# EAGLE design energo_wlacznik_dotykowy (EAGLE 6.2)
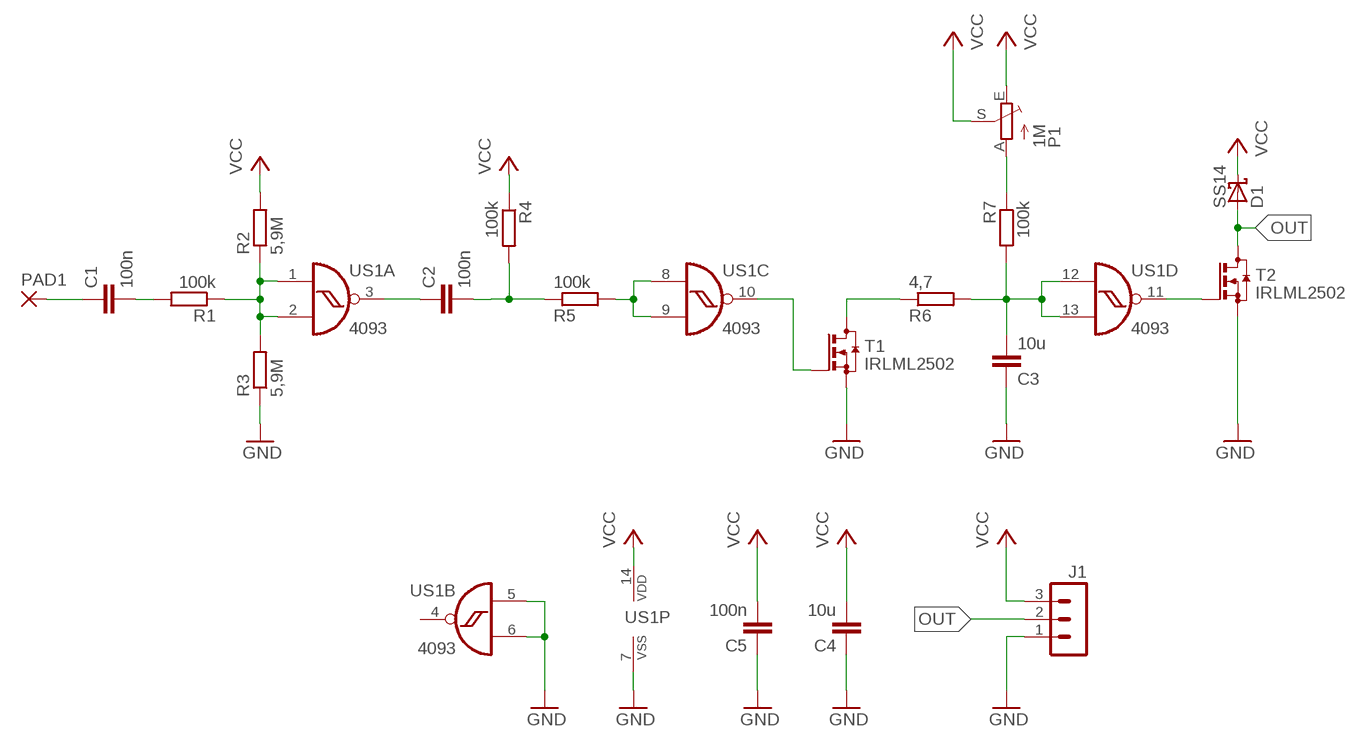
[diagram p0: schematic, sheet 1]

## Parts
C1  100n  C-EUC0805  [C0805]
C2  100n  C-EUC0805  [C0805]
C3  10u  C-EUC0805  [C0805]
C4  10u  C-EUC0805  [C0805]
C5  100n  C-EUC0805  [C0805]
D1  SS14  SCHOTTKY-DIODESMD  [SMB]
J1  MA03-1  [MA03-1]
P1  1M  TRIM_EU-CA6V  [CA6V]
PAD1  3,81/1,4  [3,81/1,4]
R1  100k  R-EU_M0805  [M0805]
R2  5,9M  R-EU_M0805  [M0805]
R3  5,9M  R-EU_M0805  [M0805]
R4  100k  R-EU_M0805  [M0805]
R5  100k  R-EU_M0805  [M0805]
R6  4,7  R-EU_M0805  [M0805]
R7  100k  R-EU_M0805  [M0805]
T1  IRLML2502  BSS123  [SOT23]
T2  IRLML2502  BSS123  [SOT23]
US1  4093  4093D  [SO14]

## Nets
GND: C3.1 C4.1 C5.1 J1.1 R3.1 T1.2(S) T2.2(S) US1.5(B:I0) US1.6(B:I1) US1.7(P:VSS)
N$1: C1.1 PAD1.1(P)
N$2: R1.1 R2.1 R3.2 US1.1(A:I0) US1.2(A:I1)
N$3: C1.2 R1.2
N$4: C2.1 US1.3(A:O)
N$5: C2.2 R4.2 R5.1
N$9: C3.2 R6.2 R7.2 US1.12(D:I0) US1.13(D:I1)
N$10: P1.A R7.1
N$11: T1.1(G) US1.10(C:O)
N$12: R6.1 T1.3(D)
N$13: T2.1(G) US1.11(D:O)
N$14: R5.2 US1.8(C:I0) US1.9(C:I1)
OUT: D1.A J1.2 T2.3(D)
VCC: C4.2 C5.2 D1.C J1.3 P1.E P1.S R2.2 R4.1 US1.14(P:VDD)
Unconnected: US1.4(B:O)

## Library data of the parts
C1-C5 = rcl:C-EU: CAPACITOR, European symbol
D1 = diode:SCHOTTKY-DIODE: Schottky Diode
J1 = con-lstb:MA03-1: PIN HEADER; OC_FARNELL: unknown; OC_NEWARK: unknown
P1 = pot:TRIM_EU-: POTENTIOMETER
PAD1 = wirepad:3,81/1,4: THROUGH-HOLE PAD
R1-R7 = rcl:R-EU_: RESISTOR, European symbol
T1 T2 = transistor-small-signal:BSS123: N-CHANNEL MOS FET
US1 = 40xx:4093: Quad 2-input NAND schmitt trigger

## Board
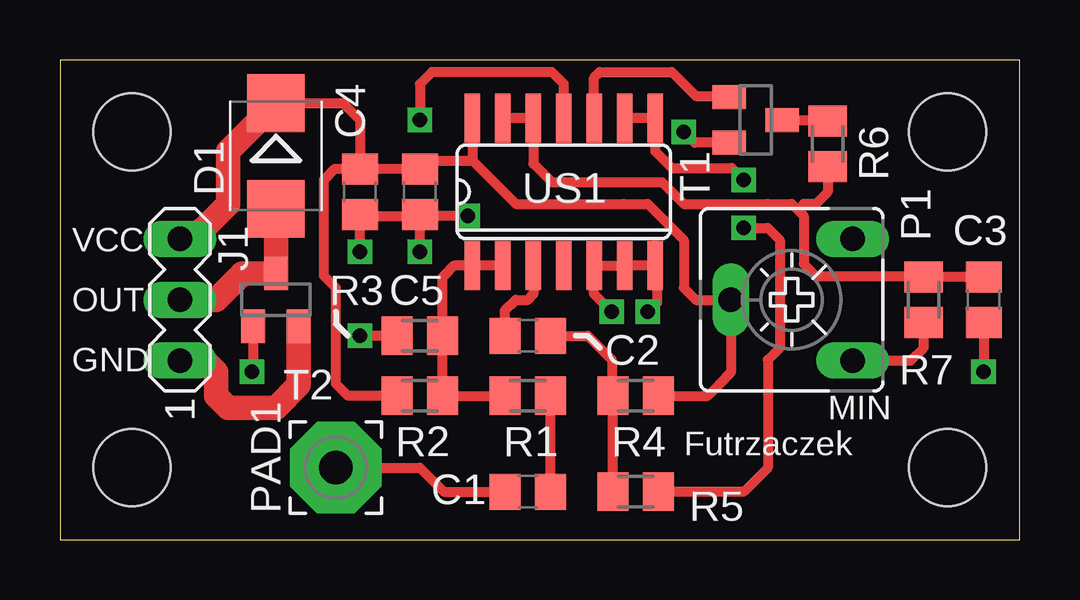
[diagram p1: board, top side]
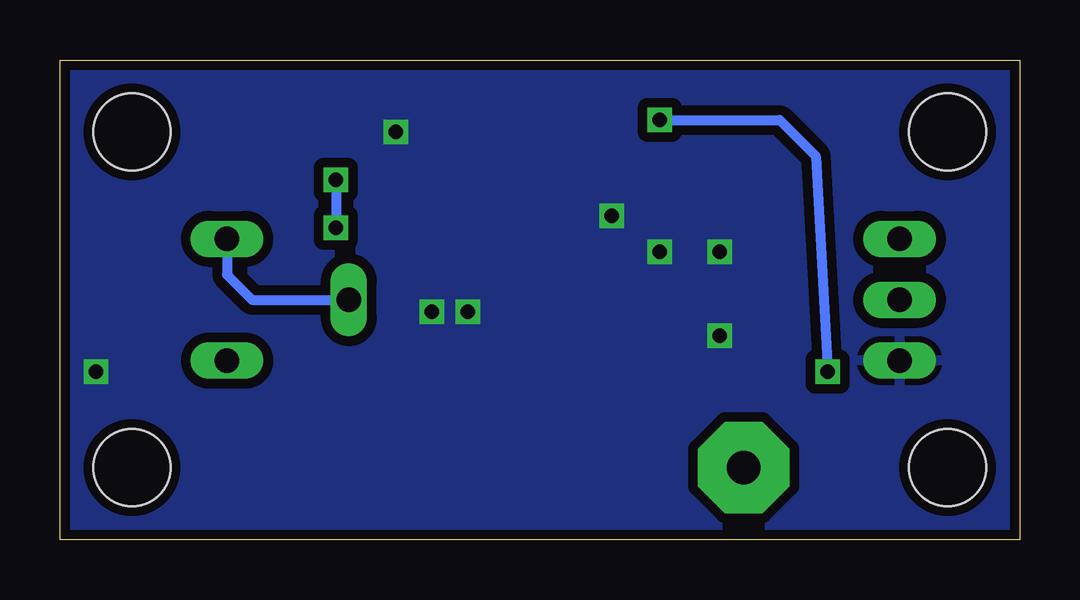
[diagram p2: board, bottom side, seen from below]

Size 40 x 20 mm. Coordinates in mm from the lower left corner, seen from the top.
Outline: 0,0 40,0 40,20 0,20 0,0
Copper layers (1*16): Top 0.035mm / dielectric 1.5mm / Bottom 0.035mm
Design rules: minimum track width 10mil, minimum drill 23mil, track to track 8mil, track to pad 8mil, pad to pad 8mil, via to via 8mil, smd to smd 8mil, copper to edge 10mil, drill to drill 8mil, minimum pad ring 10mil, minimum via ring 8mil, stop-mask expansion 4mil, vias tented up to drill 0mil, thermal gap 10mil
Holes 3.2 mm at 3,3 3,17 37,3 37,17

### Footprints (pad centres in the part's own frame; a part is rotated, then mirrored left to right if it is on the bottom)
C0805 = smd 1.3 x 1.5: 1 -0.95,0; 2 0.95,0
SMB = smd 2.4 x 2.4: A 2.2,0; C -2.2,0
MA03-1 = drill 1.016 long: 1 -2.54,0; 2 0,0; 3 2.54,0
CA6V = drill 1.016 long: A -2.54,-2.54; E 2.54,-2.54; S 0,2.54
3,81/1,4 = drill 1.397 pad 3.81 octagon: 1 0,0
M0805 = smd 1.3 x 1.6: 1 -0.95,0; 2 0.95,0
SOT23 = smd 1 x 1.4: 1 -0.95,-1.1; 2 0.95,-1.1; 3 0,1.1
SO14 = smd 0.66 x 2.032: 1 -3.81,-3.073; 2 -2.54,-3.073; 3 -1.27,-3.073; 4 0,-3.073; 5 1.27,-3.073; 6 2.54,-3.073; 7 3.81,-3.073; 8 3.81,3.073; 9 2.54,3.073; 10 1.27,3.073; 11 0,3.073; 12 -1.27,3.073; 13 -2.54,3.073; 14 -3.81,3.073

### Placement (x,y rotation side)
C1  19.5,2 0 top
C2  19.5,8.5 0 top
C3  38.5,10 90 top
C4  12.5,14.5 90 top
C5  15,14.5 90 top
D1  9,16 270 top
J1  5,10 90 top
P1  30.5,10 90 top
PAD1  11.5,3 0 top
R1  19.5,6 0 top
R2  15,6 180 top
R3  15,8.5 0 top
R4  24,6 180 top
R5  24,2 0 top
R6  32,16.5 270 top
R7  36,10 90 top
T1  29,17.5 270 top
T2  9,10 0 top
US1  21,14.5 0 top

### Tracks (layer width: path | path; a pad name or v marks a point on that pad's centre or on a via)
GND  (via drill 0.6)
  Top 0.406: 14.95,13.5 C5.1 | v15,12 15,13.5 | 15,13.5 C5.1 | US1.7 24.81,12.31 | US1.7 24.81,11.19 | v17,13.5 15.05,13.5 C5.1 | T1.2 26.45,16.55 v26,17 | C3.1 v38.5,7 | v12.5,12 12.5,13.5 | 12.5,13.5 15,13.5 | C4.1 12.5,13.5 | 22.5,11.43 US1.6 | 22.5,11.43 US1.6 | 22.5,11.43 US1.6 | v23,9.5 22.27,10.23 US1.5 22.5,11.43 | US1.7 US1.6 | v24.5,9.5 24.9,9.9 24.9,11.3 24.8,11.4 | R3.1 v12.5,8.5
  Top 1.016: T2.2 9.95,6.45 9,5.5 7,5.5 6.5,6 6.5,7 6.04,7.46 J1.1
  pour Bottom (isolate 0.406): 0,20 40,20 40,0 0,0
N$1
  Top 0.406: PAD1.1 15,3 16,2 C1.1
N$2
  Top 0.406: US1.2 US1.1 16.43,11.43 16,11 15.95,10.95 R3.2 R2.1 R1.1
N$3
  Top 0.406: C1.2 R1.2
N$4
  Top 0.406: US1.3 19.73,10.23 19.5,10 19,10 18.55,9.55 C2.1
N$5
  Top 0.406: R5.1 R4.2 23,6.05 23,7.5 22,8.5 C2.2
N$9
  Top 0.406: US1.13 US1.12 19.73,15.67 20.5,14.9 23.6,14.9 25.1,14.9 26,14 29.5,14 30.5,14 30.75,13.75 | C3.2 R7.2 | 35.95,11 R7.2 | 30.75,13.75 31,13.5 31,11.5 31.5,11 35.95,11 | 35.95,11 R7.2 | R6.2 32,14.5 31.5,14 31,14 30.75,13.75
N$10
  Top 0.406: P1.A 35.46,7.46 36,8 R7.1
N$11
  Top 0.406: US1.10 22.27,19.27 22.5,19.5 25.5,19.5 26.5,18.5 27.85,18.5 T1.1
N$12
  Top 0.406: T1.3 31.95,17.5 R6.1
N$13  (via drill 0.6)
  Top 0.254: T2.1 8.05,9.05
  Top 0.406: US1.11 21,19 20.5,19.5 15.5,19.5 15,19 v15,17.5 | T2.1 8.05,7.05 v8,7
  Bottom 0.406: v15,17.5 10,17.5 9,16.5 8.5,16 v8,7
N$14  (via drill 0.6)
  Top 0.406: US1.9 US1.8 24.81,16.19 25.5,15.5 28,15.5 v28.5,15 | v28.5,13 29.5,13 30,12.5 30,8 29.5,7.5 29.5,3 28.5,2 R5.2
  Bottom 0.406: v28.5,15 v28.5,13
OUT
  Top 1.016: J1.2 6.5,10 7.5,11 7.6,11.1 T2.3 D1.A
VCC
  Top 0.406: US1.14 17.19,15.81 | 17.19,15.81 15,15.81 C5.2 C4.2 | D1.C 11.8,18.2 12.5,17.5 C4.2 | 17.19,15.81 19,14 23.5,14 24.5,14 26,12.5 26,10.5 26.5,10 P1.S 27.96,6.96 27.5,6.5 27,6 R4.1 | R2.2 12,6 11.5,6.5 11.5,10.5 11,11 11,15 11.45,15.45 C4.2
  Top 1.016: J1.3 5.54,12.54 6.5,13.5 7,14 7,16.2 D1.C
  Bottom 0.406: P1.E 33.04,11.04 32,10 P1.S

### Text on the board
tPlace: VCC | OUT | GND | MIN | Futrzaczek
